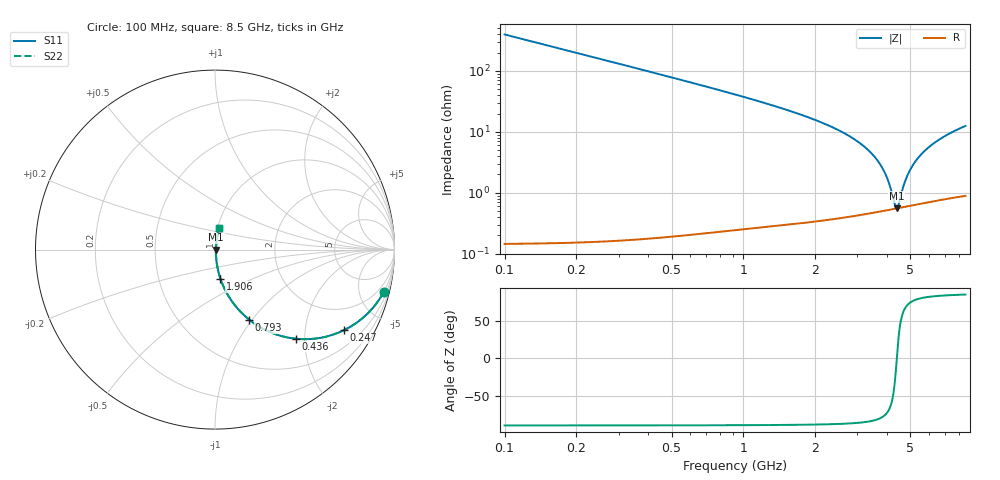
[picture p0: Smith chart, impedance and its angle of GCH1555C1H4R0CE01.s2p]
!Murata Part Number: GCH1555C1H4R0CE01
!These Parameters are Measured in Series Mode Connection
!Data Generated on Mar 13, 2026
!  o--ll--o
!Port1  Port2
!  o------o
!Operation Temp=25[degC], DC Bias Voltage=0[V]
!Freq. Start=100[MHz] Stop=9[GHz] 401[Steps]
# Hz S RI R 50
!Freq.(Hz) S11(Real) S11(Imag) S21(Real) S21(Imag) S12(Real) S12(Imag) S22(Real) S22(Imag)
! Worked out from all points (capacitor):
!   401 points, 100 MHz to 8.5 GHz, reference 50 ohm
!   read as one part in series: C = 4 pF near 142 MHz
!   lowest |Z| = 553 mohm at 4.384 GHz (marker M1)
!   series resonance near 4.387 GHz, so ESL is about 330 pH
!   S11 on the Smith chart (normalised r, x): 100 MHz: 1.00, -7.95; 247 MHz: 1.00, -3.21; 436 MHz: 1.00, -1.81; 793 MHz: 1.00, -0.97; 1.906 GHz: 1.01, -0.34; 8.5 GHz: 1.02, +0.25
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1e8  0.9404 -0.2365  0.0596 0.2365  0.0596 0.2365  0.9404 -0.2365
2.47e8  0.7202 -0.4484  0.2798 0.4484  0.2798 0.4484  0.7202 -0.4484
4.36e8  0.4492 -0.4964  0.5508 0.4964  0.5508 0.4964  0.4492 -0.4964
6.04e8  0.2946 -0.4543  0.7054 0.4543  0.7054 0.4543  0.2946 -0.4543
7.93e8  0.1912 -0.3909  0.8088 0.3909  0.8088 0.3909  0.1912 -0.3909
1.087e9  0.1069 -0.3052  0.8931 0.3052  0.8931 0.3052  0.1069 -0.3052
1.507e9  0.0536 -0.2188  0.9464 0.2188  0.9464 0.2188  0.0536 -0.2188
1.906e9  0.0306 -0.1627  0.9694 0.1627  0.9694 0.1627  0.0306 -0.1627
2.914e9  0.00975 -0.0745  0.9903 0.0745  0.9903 0.0745  0.00975 -0.0745
3.418e9  0.00661 -0.0447  0.9934 0.0447  0.9934 0.0447  0.00661 -0.0447
3.796e9  0.00561 -0.0257  0.9944 0.0257  0.9944 0.0257  0.00561 -0.0257
4.048e9  0.00539 -0.0142  0.9946 0.0142  0.9946 0.0142  0.00539 -0.0142
4.3e9  0.00544 -0.00353  0.9946 0.00353  0.9946 0.00353  0.00544 -0.00353
4.384e9  0.0055 -0.000111  0.9945 0.000111  0.9945 0.000111  0.0055 -0.000111
4.447e9  0.00557 0.00241  0.9944 -0.00241  0.9944 -0.00241  0.00557 0.00241
4.72e9  0.00599 0.0129  0.994 -0.0129  0.994 -0.0129  0.00599 0.0129
4.93e9  0.00644 0.0206  0.9936 -0.0206  0.9936 -0.0206  0.00644 0.0206
5.266e9  0.00737 0.0322  0.9926 -0.0322  0.9926 -0.0322  0.00737 0.0322
5.707e9  0.0089 0.0465  0.9911 -0.0465  0.9911 -0.0465  0.0089 0.0465
6.316e9  0.0115 0.0647  0.9885 -0.0647  0.9885 -0.0647  0.0115 0.0647
7.114e9  0.0155 0.0866  0.9845 -0.0866  0.9845 -0.0866  0.0155 0.0866
8.5e9  0.0238 0.1208  0.9762 -0.1208  0.9762 -0.1208  0.0238 0.1208
